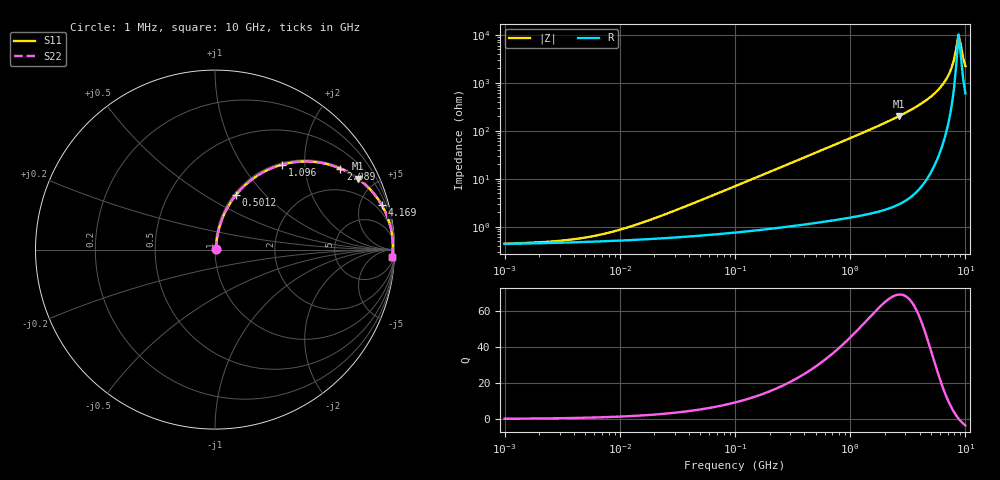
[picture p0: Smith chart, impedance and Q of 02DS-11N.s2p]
# MHz S MA R 50
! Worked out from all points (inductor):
!   201 points, 1 MHz to 10 GHz, reference 50 ohm
!   read as one part in series: L = 11 nH near 25.12 MHz
!   highest Q = 69.1 at 2.63 GHz (marker M1), where L = 12.1 nH
!   self-resonance near 8.71 GHz
!   S11 on the Smith chart (normalised r, x): 1 MHz: 1.01, +0.00; 501.2 MHz: 1.02, +0.70; 1.096 GHz: 1.03, +1.54; 2.089 GHz: 1.05, +3.06; 4.169 GHz: 1.14, +7.45; 10 GHz: 13, -43
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1  0.004385 9.0  0.9957 -0.0  0.9957 -0.0  0.004385 9.0
4.7863  0.005774 34.6  0.9953 -0.2  0.9953 -0.2  0.005774 34.6
9.54993  0.008288 52.0  0.9949 -0.4  0.9949 -0.4  0.008288 52.0
21.8776  0.01605 68.7  0.9943 -0.9  0.9943 -0.9  0.01605 68.7
104.713  0.07205 79.9  0.9899 -4.1  0.9899 -4.1  0.07205 79.9
229.087  0.1553 77.7  0.9788 -8.9  0.9788 -8.9  0.1553 77.7
478.63  0.3118 69.8  0.9392 -18.2  0.9392 -18.2  0.3118 69.8
501.187  0.325 69.1  0.9347 -19.0  0.9347 -19.0  0.325 69.1
758.578  0.4622 61.0  0.8748 -27.5  0.8748 -27.5  0.4622 61.0
1096.48  0.6041 51.7  0.7844 -37.2  0.7844 -37.2  0.6041 51.7
2089.3  0.8315 32.9  0.5431 -56.2  0.5431 -56.2  0.8315 32.9
2187.76  0.8443 31.6  0.5235 -57.6  0.5235 -57.6  0.8443 31.6
2630.27  0.8891 26.4  0.445 -62.8  0.445 -62.8  0.8891 26.4
4168.69  0.9613 15.0  0.2582 -74.0  0.2582 -74.0  0.9613 15.0
5754.4  0.9846 8.1  0.141 -79.7  0.141 -79.7  0.9846 8.1
6918.31  0.9903 4.5  0.07846 -80.6  0.07846 -80.6  0.9903 4.5
7585.78  0.9913 2.7  0.04822 -78.2  0.04822 -78.2  0.9913 2.7
7943.28  0.9913 1.9  0.03347 -74.1  0.03347 -74.1  0.9913 1.9
8317.64  0.9911 1.0  0.01947 -62.3  0.01947 -62.3  0.9911 1.0
8709.64  0.9906 0.1  0.009707 -14.0  0.009707 -14.0  0.9906 0.1
9549.93  0.9886 -1.6  0.02971 66.7  0.02971 66.7  0.9886 -1.6
10000  0.9872 -2.4  0.04421 71.9  0.04421 71.9  0.9872 -2.4
